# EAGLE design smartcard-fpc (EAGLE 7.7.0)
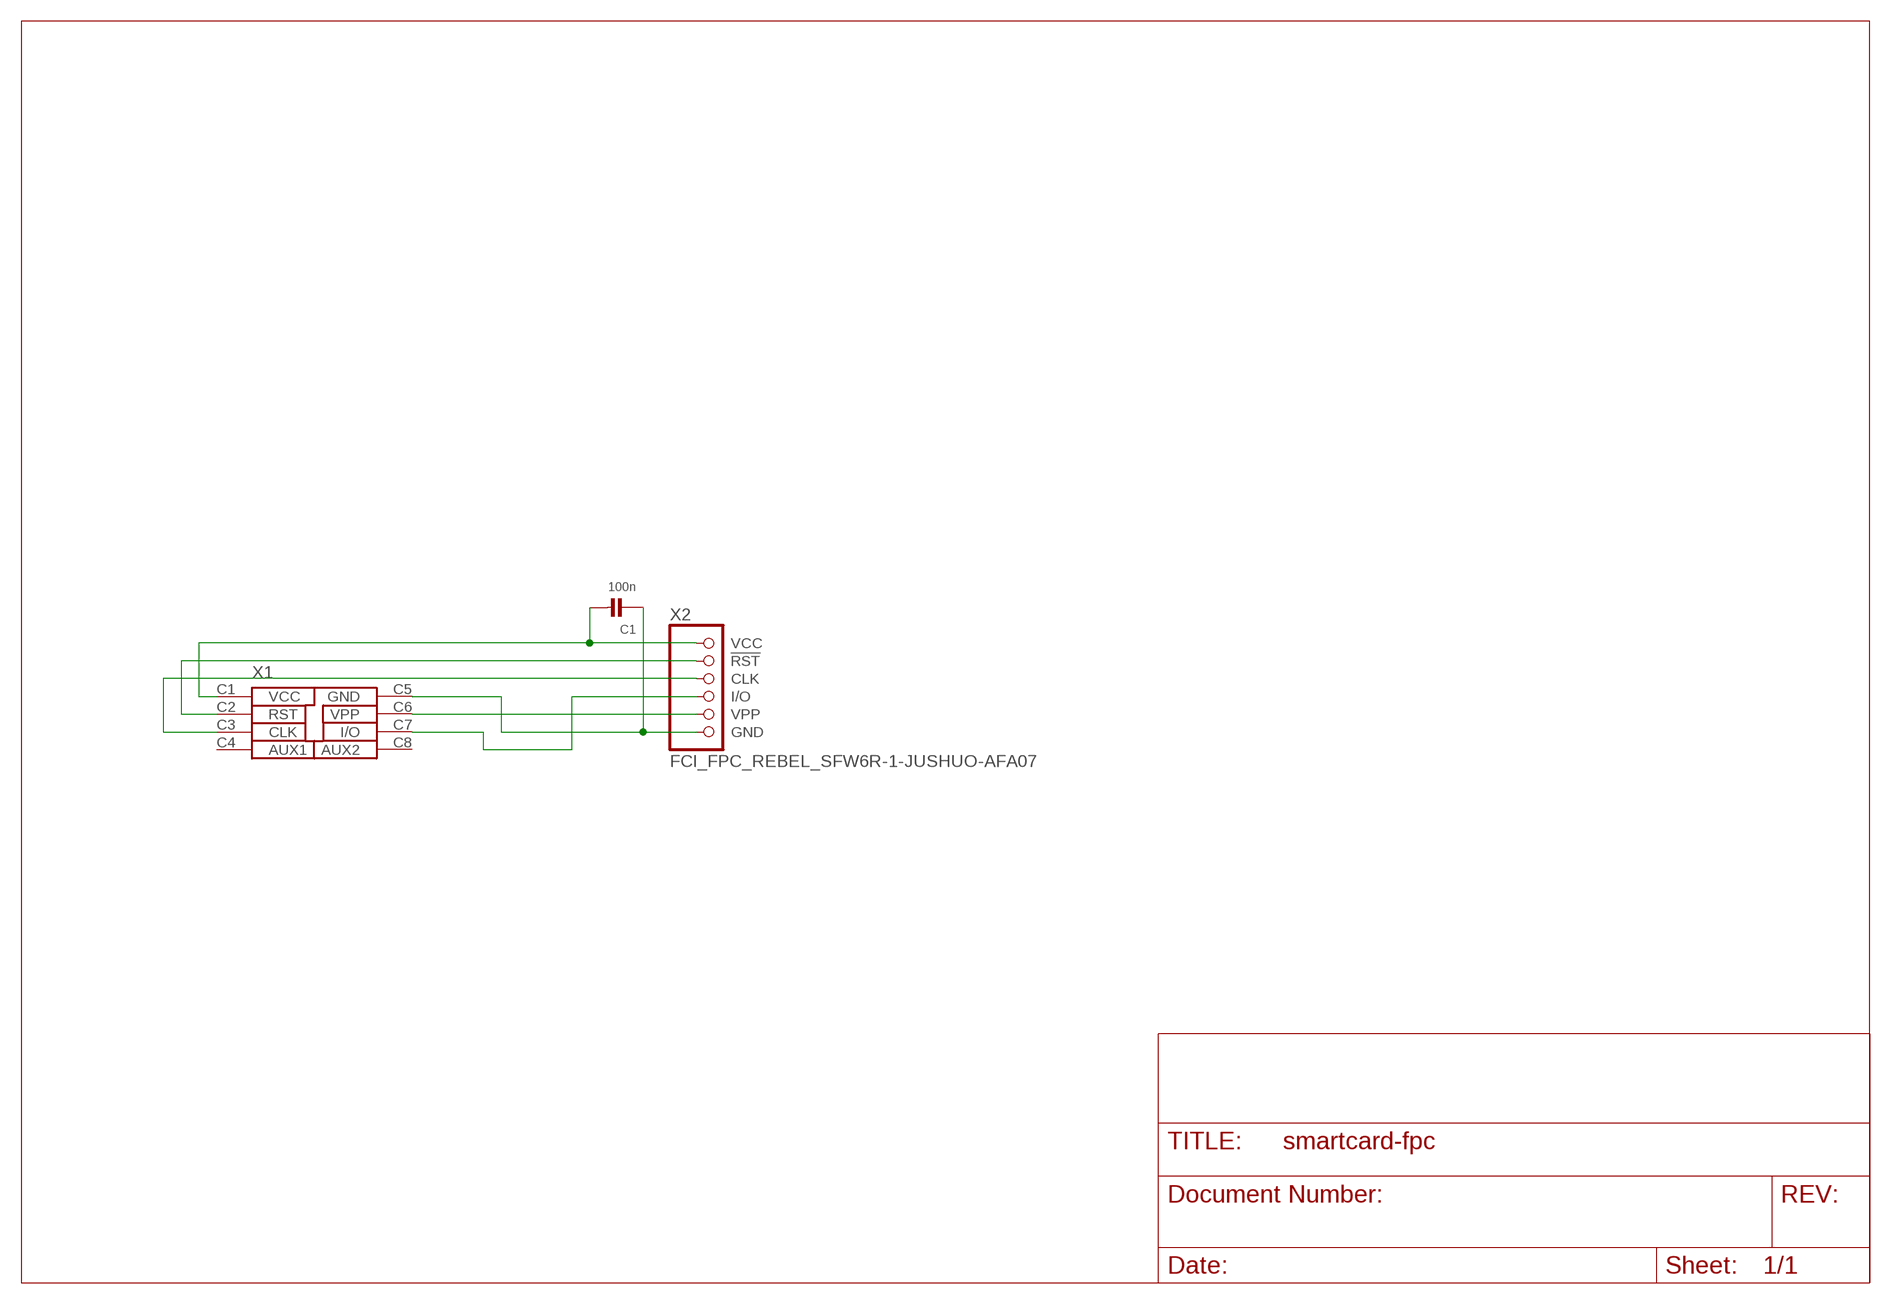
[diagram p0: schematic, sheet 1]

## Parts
C1  100n  CAP_CERAMIC_0603  [_0603]
X1  SMARTCARD  [ISO7816_CARD]
X2  FCI_FPC_REBEL_SFW6R-1-JUSHUO-AFA07  [FPC_JUSHUO_AFA07-S06]

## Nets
CLK: X1.C3(CLK) X2.3(CLK)
GND: C1.1 X1.C5(GND) X2.6(GND)
IO: X1.C7(I/O) X2.4(I/O)
RST: X1.C2(RST) X2.2(!RST)
VCC: C1.2 X1.C1(VCC) X2.1(VCC)
VPP: X1.C6(VPP) X2.5(VPP)
Unconnected: X1.C4(AUX1) X1.C8(AUX2)

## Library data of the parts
C1 = rc-sysmocom:CAP_CERAMIC: Ceramic Capacitors
X1 = iso7816-card:SMARTCARD: ISO 7916 SMart Card
X2 = laforge:FCI_FPC_REBEL_SFW6R-1

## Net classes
0 default: width 0.6 mm

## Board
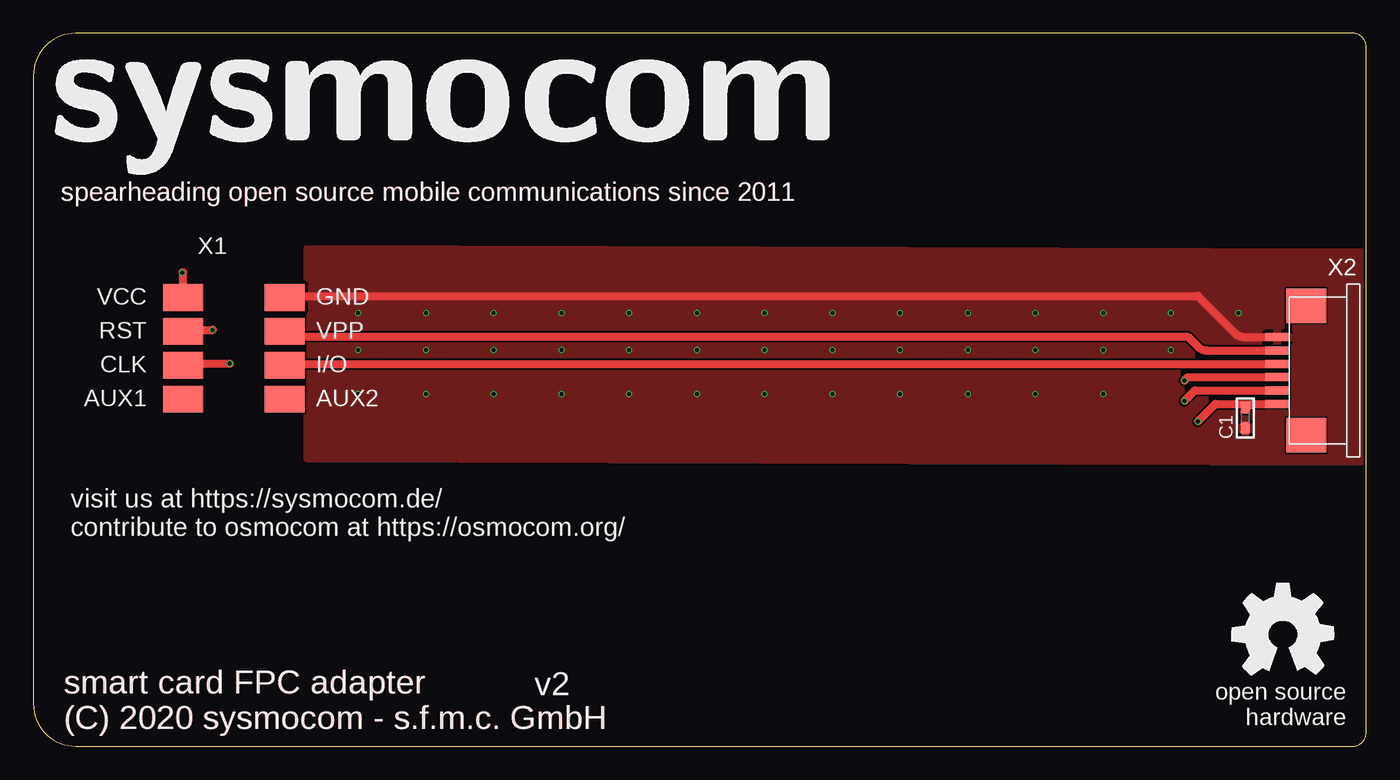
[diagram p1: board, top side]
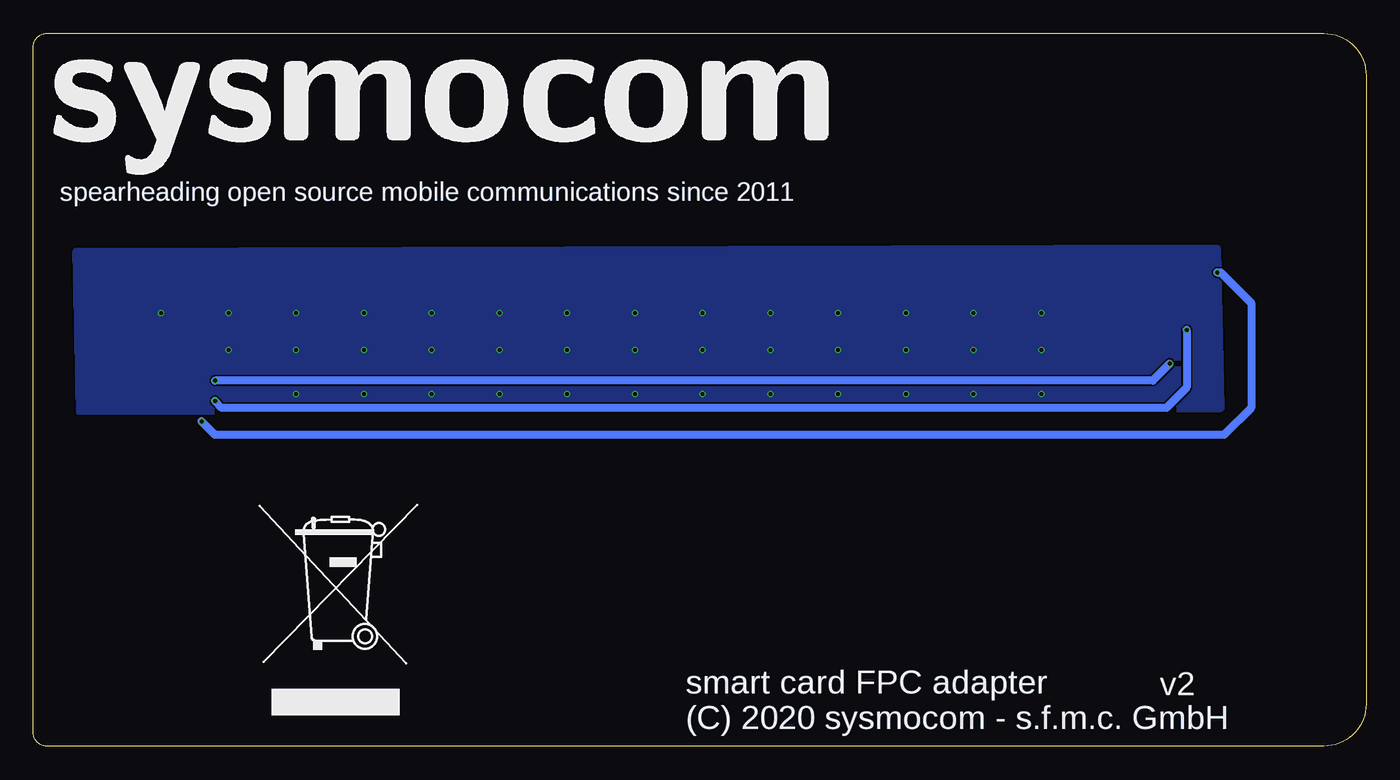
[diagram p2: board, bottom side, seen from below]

Size 100 x 53.5 mm. Coordinates in mm from the lower left corner, seen from the top.
Outline: 0,50.32 0,3.18 arc90 3.18,0 99,0 arc90 100,1 100,52.5 arc90 99,53.5 3.18,53.5 arc90 0,50.32
Copper layers (1*16): Top 0.035mm / dielectric 1.6mm / Bottom 0.035mm
Design rules "jlcpcb-2layers *": minimum track width 5mil, minimum drill 0.3mm, track to track 5mil, track to pad 5mil, pad to pad 5mil, via to via 5mil, smd to smd 5mil, copper to edge 0.2mm, drill to drill 6mil, minimum pad ring 10mil, minimum via ring 3mil, stop-mask expansion 4mil, vias tented up to drill 0.4mm, thermal gap 10mil

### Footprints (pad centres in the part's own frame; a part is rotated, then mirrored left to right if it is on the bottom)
_0603 = smd 0.9 x 0.8: 1 -0.762,0; 2 0.762,0
ISO7816_CARD = smd 3 x 2: C1 -31.55,6.92; C2 -31.55,4.38; C3 -31.55,1.85; C4 -31.55,-0.7; C5 -23.93,6.92; C6 -23.93,4.38; C7 -23.93,1.85; C8 -23.93,-0.7
FPC_JUSHUO_AFA07-S06 = smd 0.6 x 1.8: 1 -2.5,0.9; 2 -1.5,0.9; 3 -0.5,0.9; 4 0.5,0.9; 5 1.5,0.9; 6 2.5,0.9 | smd 2.6 x 3: M1 -4.85,-1.27; M2 4.85,-1.27

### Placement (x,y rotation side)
C1  90.93,24.64 90 top
U$1  [WEEE_BIN_TOP]  77.72,11.43 0 bottom
U$2  [WEEE_BIN]  77.72,8.89 0 bottom
U$3  [OSHW_8MM]  93.73,8.38 0 top
U$4  [SYSMOCOM-58]  1.52,42.93 0 top
U$5  [SYSMOCOM-58-TOP]  1.52,42.93 0 top
U$6  [SYSMOCOM-58-BOT]  40.39,42.93 0 top
U$7  [SYSMOCOM-58-BPLACE]  40.39,42.93 0 top
X1  42.8,26.75 0 top
X2  94.23,28.19 90 top

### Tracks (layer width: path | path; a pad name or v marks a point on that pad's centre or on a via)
CLK  (via drill 0.3)
  Top 0.6: X1.C3 11.35,28.7 v14.73,28.7 | v86.36,27.43 86.62,27.69 X2.3
  Bottom 0.6: v14.73,28.7 16,27.43 v86.36,27.43
GND  (via drill 0.3)
  Top 0.6: X1.C5 arc-45 19.14,33.78 87.38,33.78 90.17,30.99 arc45 90.88,30.69 X2.6
  other vias: 24.38,32.51 24.38,26.42 24.38,29.72 29.46,32.51 34.54,32.51 39.62,32.51 44.7,32.51 49.78,32.51 54.86,32.51 59.94,32.51 65.02,32.51 70.1,32.51 75.18,32.51 80.26,32.51 85.34,32.51 90.42,32.51 29.46,29.72 34.54,29.72 39.62,29.72 44.7,29.72 49.78,29.72 54.86,29.72 59.94,29.72 65.02,29.72 70.1,29.72 75.18,29.72 80.26,29.72 85.34,29.72 29.46,26.42 34.54,26.42 39.62,26.42 44.7,26.42 49.78,26.42 54.86,26.42 59.94,26.42 65.02,26.42 70.1,26.42 75.18,26.42 80.26,26.42
  pour Top: 20.57,37.34 99.57,37.08 99.57,21.34 20.57,21.59
  pour Bottom: 11.18,37.34 96.77,37.08 96.52,25.15 10.92,25.4
IO
  Top 0.6: X1.C7 arc-45 19.1,28.69 X2.4
RST  (via drill 0.3)
  Top 0.6: X1.C2 arc-90 11.36,31.24 v13.46,31.24 | v86.36,25.91 87.15,26.69 X2.2
  Bottom 0.6: v13.46,31.24 13.46,26.92 14.99,25.4 85.85,25.4 v86.36,25.91
VCC  (via drill 0.3)
  Top 0.6: X1.C1 11.25,35.56 v11.18,35.56 | v87.38,24.38 88.69,25.69 91.48,25.69 | C1.2 91.48,25.69 | 91.48,25.69 X2.1
  Bottom 0.6: v11.18,35.56 10.92,35.56 8.64,33.27 8.64,25.4 10.67,23.37 86.36,23.37 v87.38,24.38
VPP
  Top 0.6: X1.C6 18.97,31.03 arc45 19.68,30.73 86.61,30.73 87.36,29.99 arc45 88.07,29.69 X2.5

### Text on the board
Top: spearheading open source mobile communications since 2011 | smart card FPC adapter / (C) 2020 sysmocom - s.f.m.c. GmbH
Bottom: spearheading open source mobile communications since 2011 | smart card FPC adapter / (C) 2020 sysmocom - s.f.m.c. GmbH
tPlace: spearheading open source mobile communications since 2011 | visit us at https://sysmocom.de/ / contribute to osmocom at https://osmocom.org/
bPlace: spearheading open source mobile communications since 2011
tNames: smart card FPC adapter / (C) 2020 sysmocom - s.f.m.c. GmbH
bNames: smart card FPC adapter / (C) 2020 sysmocom - s.f.m.c. GmbH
